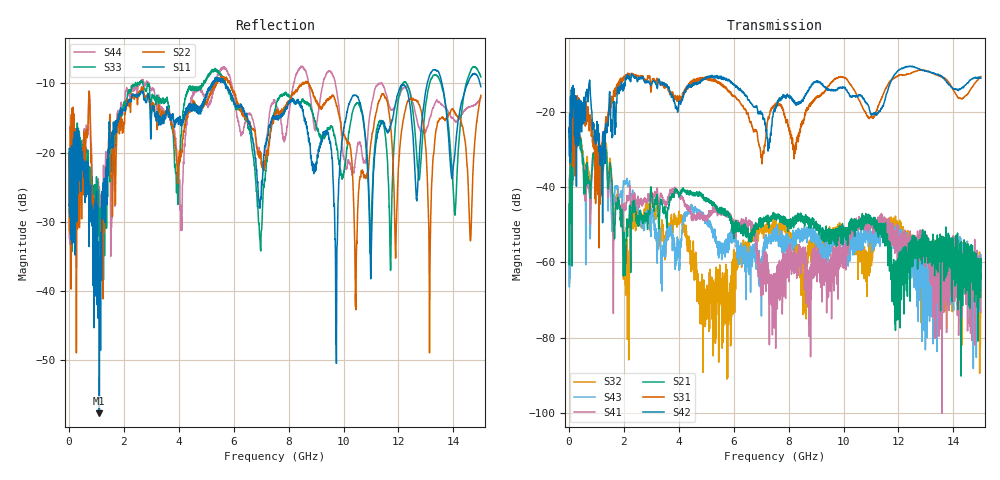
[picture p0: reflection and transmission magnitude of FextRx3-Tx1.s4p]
! FILE: N:\QM 2007\Prüfprotokolle\Highspeed\Konfektionierte Ltg\L45593-D106\D30\8216\0002\Fext\FextRx3-Tx1.s4p
# MHz S DB R 50.00
! FREQ  S11  S12  S13  S14
!  S21  S22  S23  S24
!  S31  S32  S33  S34
!  S41  S42  S43  S44
!  DB  ANG  DB  ANG  DB  ANG  DB  ANG
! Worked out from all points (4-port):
!   2999 points, 10 MHz to 15 GHz, reference 50 ohm
!   strongest paths, dB at 10 MHz, 3.755 GHz, 7.505 GHz, 11.26 GHz, 15 GHz:
!     S42: -25.5, -15.5, -19.7, -20.4, -11.2
!     S31: -24.5, -15.7, -18.1, -18.6, -10.7
!     S21: -44.5, -42.0, -47.8, -50.6, -61.6
!     S41: -58.9, -40.8, -77.0, -51.0, -73.2
!     S43: -48.2, -52.6, -52.0, -51.6, -67.2
!     S32: -57.4, -51.9, -50.4, -49.2, -63.6
!   lowest |S11| = -57.7 dB at 1.11 GHz (marker M1), VSWR 1.00, Z = 50 - j0.125 ohm
!   |S11| at or under -10 dB: start of sweep to 5.214 GHz; 5.693 GHz to 13.05 GHz (7.356 GHz wide, 78.5 % of centre); 13.58 GHz to 14.52 GHz (937.8 MHz wide, 6.67 % of centre)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
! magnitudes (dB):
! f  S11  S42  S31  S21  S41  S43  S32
! 10 MHz  -19.4  -25.5  -24.5  -44.5  -58.9  -48.2  -57.4
! 280 MHz  -18.3  -26.0  -18.2  -25.6  -26.1  -26.3  -25.1
! 1.11 GHz  -57.7  -26.5  -34.3  -34.1  -35.3  -35.5  -32.9
! 5.06 GHz  -11.3  -10.7  -11.2  -43.3  -48.2  -49.3  -66.7
! 9.72 GHz  -47.6  -14.3  -11.3  -52.5  -56.3  -54.9  -53.9
! 10.45 GHz  -11.7  -15.9  -15.2  -50.5  -50.5  -55.2  -57.9
! 15 GHz  -10.5  -11.2  -10.7  -61.6  -73.2  -67.2  -63.6
